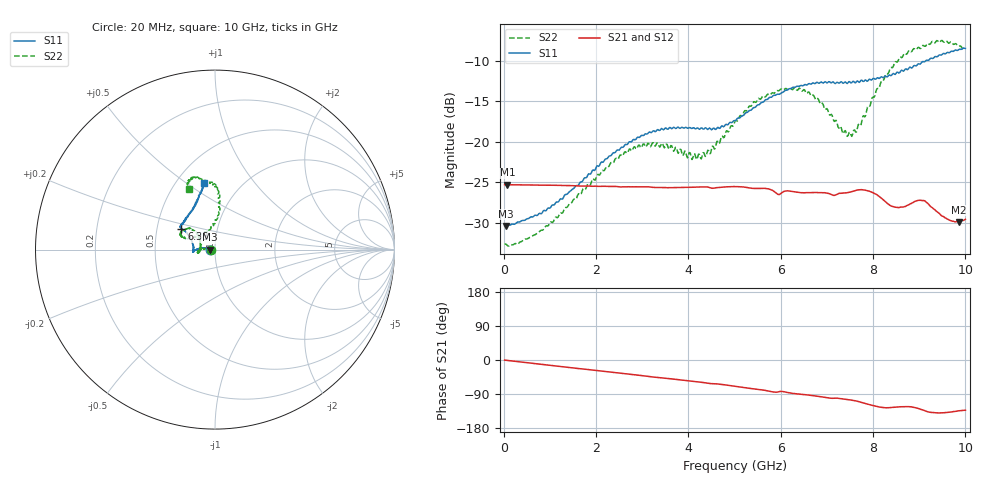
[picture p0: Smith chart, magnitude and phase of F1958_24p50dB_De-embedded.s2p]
! Integrated Device Technology
! Corporate Headquarters
! 6024 Silver Creek Valley Road
! San Jose, CA 95138  USA
! Phone:  1-408-284-8200
! Toll Free:  1-800-223-1366
! Webpage:  http://www.idt.com/
! Timing and RF Division
! 515 Groton Road, Suite 102
! Westford, MA 01886-6024
! Device:  F1958
! Description: 7-bit 0.25 dB Digital Step Attenuator
! Frequency:  0.001 -  6.000 GHz
! Package:  4x4 mm Thin QFN Plastic Package: 24 pin
! Ports:  2 RF, 12 DC
!  Pin  1  = D0
!  Pin  2  = VDD
!  Pin  3  = VMODE
!  Pin  4  = GND
!  Pin  5  = RF1  =  Port 1
!  Pin  6  = GND
!  Pin  7  = GND
!  Pin  8  = GND
!  Pin  9  = GND
!  Pin 10  = GND
!  Pin 11  = GND
!  Pin 12  = GND
!  Pin 13  = GND
!  Pin 14  = RF2  =  Port 2
!  Pin 15  = GND
!  Pin 16  = LE
!  Pin 17  = CLK
!  Pin 18  = DATA
!  Pin 19  = D6
!  Pin 20  = D5
!  Pin 21  = D4
!  Pin 22  = D3
!  Pin 23  = D2
!  Pin 24  = D1
! State:  98
! Atten State:  24.50 dB
! Voltage:  +3.30 Volts
! Current:  0.258 mA
! Data:  The device was measured on a F1958 evaluation board which has
!  individual transmission lines to the RF pins.  Data was collected
!  using a calibrated network analyzer.  The evaluation board was
!  de-embedded using Automatic Fixture Removal (AFR).
!  The reference plane is the edge of the package pin.
! Misc:
!  Action Tracker AT0419
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# GHz S dB R 50
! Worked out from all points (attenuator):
!   500 points, 20 MHz to 10 GHz, reference 50 ohm
!   highest |S21| = -25.29 dB at 80 MHz (marker M1); lowest = -29.9 dB at 9.86 GHz (marker M2)
!   lowest |S11| = -30.4 dB at 40 MHz (marker M3), VSWR 1.06, Z = 47.1 - j0.046 ohm
!   |S11| at or under -10 dB: start of sweep to 9.14 GHz
!   |S22| runs from -32.9 to -7.5 dB; largest |S21 - S12| = 0.0003
!   S11 on the Smith chart (normalised r, x): 20 MHz: 0.94, -0.00; 6.38 GHz: 0.67, +0.16; 10 GHz: 0.68, +0.59
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0.02  -30.36 -178.9  -25.30 -0.3  -25.29 -0.3  -32.65 -178.8
0.04  -30.38 -179.1  -25.30 -0.6  -25.29 -0.6  -32.60 -178.3
0.08  -30.30 179.5  -25.29 -1.2  -25.29 -1.1  -32.80 -178.6
0.84  -28.70 171.4  -25.35 -11.7  -25.35 -11.7  -30.90 173.1
1.7  -24.92 171.7  -25.47 -23.5  -25.46 -23.4  -26.06 172.3
2.62  -20.40 177.6  -25.56 -35.9  -25.54 -36.0  -21.24 -178.7
3.36  -18.58 -175.2  -25.65 -46.3  -25.64 -46.5  -20.46 -168.7
4.24  -18.46 -178.6  -25.59 -58.1  -25.60 -58.2  -21.56 169.6
4.5  -18.51 175.5  -25.72 -62.3  -25.74 -62.3  -20.94 152.1
5.02  -17.38 161.1  -25.52 -69.5  -25.53 -69.5  -17.38 138.6
5.58  -15.14 150.8  -25.75 -78.6  -25.77 -78.5  -14.64 140.2
6.38  -13.16 148.2  -26.24 -89.9  -26.26 -89.8  -13.53 155.1
6.68  -12.79 146.7  -26.27 -93.7  -26.29 -93.6  -14.30 157.8
7.5  -12.61 138.2  -26.22 -105.2  -26.21 -105.1  -18.81 120.1
7.68  -12.57 135.3  -25.94 -109.5  -25.94 -109.5  -17.88 100.2
7.92  -12.26 129.0  -26.10 -117.6  -26.09 -117.7  -15.68 88.9
8.34  -11.78 119.0  -27.72 -125.9  -27.74 -126.0  -11.44 84.1
8.7  -11.01 112.3  -27.99 -122.8  -27.96 -122.8  -9.11 90.2
9.02  -10.41 107.7  -27.22 -129.5  -27.24 -129.6  -8.49 97.7
9.26  -9.67 104.6  -28.05 -138.3  -28.04 -138.3  -7.76 102.6
9.86  -8.61 99.7  -29.90 -134.1  -29.87 -133.9  -8.21 112.4
10  -8.48 99.7  -29.57 -132.6  -29.58 -132.5  -8.66 113.6
